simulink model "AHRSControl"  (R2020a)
settings: Solver=FixedStepDiscrete  StartTime=0.0  StopTime=10.0  FixedStep=0.01  RelTol=1e-3  EnableMultiTasking=on
model workspace (MAT data in the model file):
  Ts : Simulink.Parameter (value not decoded)
symbols that are objects in the model workspace (value not decoded): Ts
undefined symbols (not defined in the file or in its folder): DiscIntNeverNeededParam
libraries: simulink x3, HeliLibrary_New x3

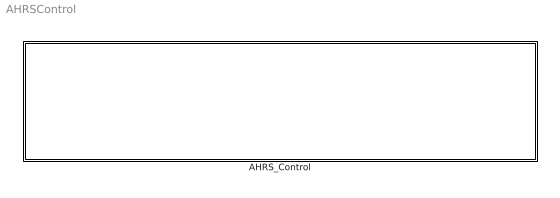
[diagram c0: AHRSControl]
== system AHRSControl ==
  AHRS_Control : Subsystem  TreatAsAtomicUnit=on

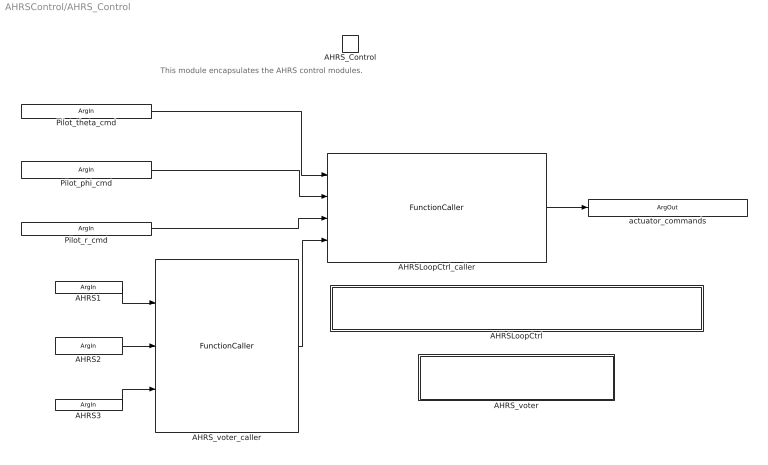
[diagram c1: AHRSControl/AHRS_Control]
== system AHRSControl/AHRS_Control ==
  note: This module encapsulates the AHRS control modules.
  AHRS_Control : TriggerPort  TriggerType=function-call  IsSimulinkFunction=on  FunctionName=AHRS_Control  FunctionVisibility=scoped  VariantControl=Variant  PortDimensions=1
  AHRSLoopCtrl : Subsystem  TreatAsAtomicUnit=on
  AHRSLoopCtrl_caller : FunctionCaller  FunctionPrototype=actuator_commands = AHRSLoopCtrl(Pilot_theta_cmd,Pilot_phi_cmd,Pilot_r_cmd,voted_fb)
  AHRS_voter : Subsystem  TreatAsAtomicUnit=on
  AHRS_voter_caller : FunctionCaller  FunctionPrototype=voted_fb = AHRS_voter(AHRS1,AHRS2,AHRS3)
  Pilot_theta_cmd : ArgIn  OutMin=-32768  OutMax=32767  OutDataTypeStr=int16  ArgumentName=Pilot_theta_cmd
  Pilot_phi_cmd : ArgIn  Port=2  OutMin=-32768  OutMax=32767  OutDataTypeStr=int16  ArgumentName=Pilot_phi_cmd
  Pilot_r_cmd : ArgIn  Port=3  OutMin=-32768  OutMax=32767  OutDataTypeStr=int16  ArgumentName=Pilot_r_cmd
  AHRS1 : ArgIn  Port=4  OutDataTypeStr=Bus: AHRS_Bus  ArgumentName=AHRS1
  AHRS2 : ArgIn  Port=5  OutDataTypeStr=Bus: AHRS_Bus  ArgumentName=AHRS2
  AHRS3 : ArgIn  Port=6  OutDataTypeStr=Bus: AHRS_Bus  ArgumentName=AHRS3
  actuator_commands : ArgOut  PortDimensions=3  ArgumentName=actuator_commands
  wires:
  AHRS3/1 -> AHRS_voter_caller/3
  AHRS1/1 -> AHRS_voter_caller/1
  AHRS2/1 -> AHRS_voter_caller/2
  Pilot_theta_cmd/1 -> AHRSLoopCtrl_caller/1
  Pilot_r_cmd/1 -> AHRSLoopCtrl_caller/3
  AHRS_voter_caller/1 -> AHRSLoopCtrl_caller/4
  AHRSLoopCtrl_caller/1 -> actuator_commands/1
  Pilot_phi_cmd/1 -> AHRSLoopCtrl_caller/2

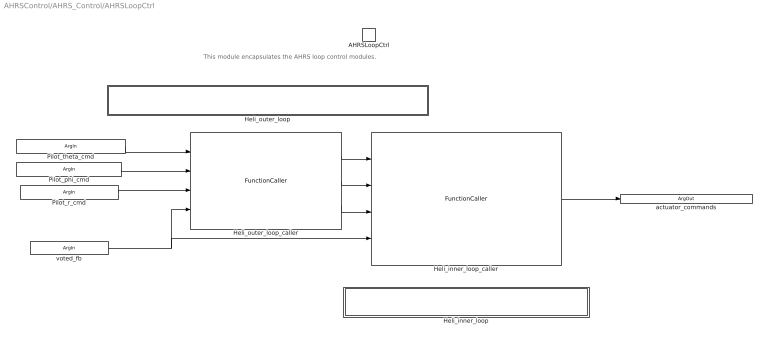
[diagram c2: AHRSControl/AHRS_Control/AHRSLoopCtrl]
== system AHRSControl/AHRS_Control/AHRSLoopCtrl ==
  note: This module encapsulates the AHRS loop control modules.
  AHRSLoopCtrl : TriggerPort  TriggerType=function-call  IsSimulinkFunction=on  FunctionName=AHRSLoopCtrl  FunctionVisibility=scoped  VariantControl=Variant  PortDimensions=1
  Heli_inner_loop : Subsystem  TreatAsAtomicUnit=on
  Heli_inner_loop_caller : FunctionCaller  FunctionPrototype=actuator_commands = Heli_inner_loop(theta_cmd,phi_cmd,r_cmd,voted_fb)
  Heli_outer_loop : Subsystem  TreatAsAtomicUnit=on
  Heli_outer_loop_caller : FunctionCaller  FunctionPrototype=[theta_cmd,phi_cmd,r_cmd] = Heli_outer_loop(Pilot_theta_cmd,Pilot_phi_cmd,Pilot_r_cmd,voted_fb)
  Pilot_theta_cmd : ArgIn  OutMin=-32768  OutMax=32767  OutDataTypeStr=int16  ArgumentName=Pilot_theta_cmd
  Pilot_phi_cmd : ArgIn  Port=2  OutMin=-32768  OutMax=32767  OutDataTypeStr=int16  ArgumentName=Pilot_phi_cmd
  Pilot_r_cmd : ArgIn  Port=3  OutMin=-32768  OutMax=32767  OutDataTypeStr=int16  ArgumentName=Pilot_r_cmd
  voted_fb : ArgIn  Port=4  OutMin=-180  OutMax=180  PortDimensions=5  ArgumentName=voted_fb
  actuator_commands : ArgOut  PortDimensions=3  ArgumentName=actuator_commands
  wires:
  Pilot_phi_cmd/1 -> Heli_outer_loop_caller/2
  Heli_outer_loop_caller/3 -> Heli_inner_loop_caller/3
  Heli_outer_loop_caller/1 -> Heli_inner_loop_caller/1
  Heli_inner_loop_caller/1 -> actuator_commands/1
  Heli_outer_loop_caller/2 -> Heli_inner_loop_caller/2
  voted_fb/1 -> Heli_outer_loop_caller/4, Heli_inner_loop_caller/4
  Pilot_r_cmd/1 -> Heli_outer_loop_caller/3
  Pilot_theta_cmd/1 -> Heli_outer_loop_caller/1

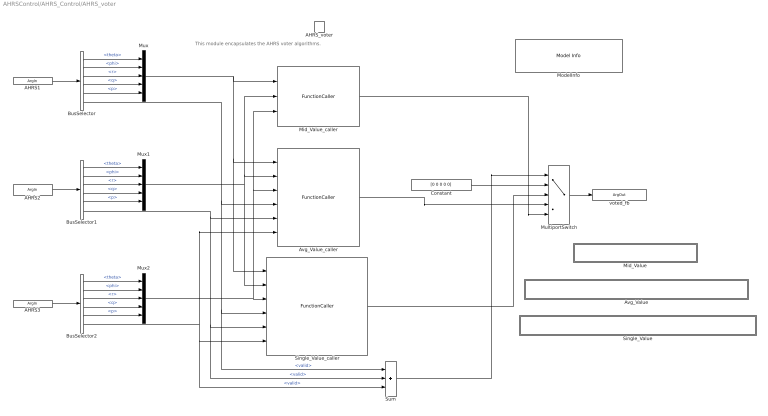
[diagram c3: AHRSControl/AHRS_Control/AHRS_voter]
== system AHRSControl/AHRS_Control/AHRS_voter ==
  note: This module encapsulates the AHRS voter algorithms.
  AHRS_voter : TriggerPort  TriggerType=function-call  IsSimulinkFunction=on  FunctionName=AHRS_voter  FunctionVisibility=scoped  VariantControl=Variant  PortDimensions=1
  Avg_Value : Subsystem  TreatAsAtomicUnit=on  RTWFcnName=Avg_Value
  Avg_Value_caller : FunctionCaller  FunctionPrototype=Avg_Value = Avg_Value(AHRS1,AHRS2,AHRS3,AHRS1_Valid,AHRS2_Valid,AHRS3_Valid)
  BusSelector : BusSelector  OutputSignals=theta,phi,r,q,p,valid
  BusSelector1 : BusSelector  OutputSignals=theta,phi,r,q,p,valid
  BusSelector2 : BusSelector  OutputSignals=theta,phi,r,q,p,valid
  Constant : Constant  Value=[0 0 0 0 0]
  Mid_Value : Subsystem  TreatAsAtomicUnit=on  RTWFcnName=Mid_Value
  Mid_Value_caller : FunctionCaller  FunctionPrototype=Mid_Value = Mid_Value(AHRS1,AHRS2,AHRS3)
  ModelInfo : simulink/Model-Wide Utilities/Model Info  Frame=on  DisplayStringWithTags=|  HorizontalTextAlignment=Center  LeftAlignmentValue=0.5
      | Model Name: %<ModelName>
      | Model Version: %<ModelVersion>
      | Last Modified: %<LastModificationDate>
      | 
      | Copyright 2016 The MathWorks, Inc.
  MultiportSwitch : MultiPortSwitch  DataPortOrder=Zero-based contiguous  Inputs=4  DiagnosticForDefault=None  zeroidx=on
  Mux : Mux  Inputs=5
  Mux1 : Mux  Inputs=5
  Mux2 : Mux  Inputs=5
  Single_Value : Subsystem  TreatAsAtomicUnit=on  RTWFcnName=Single_Value
  Single_Value_caller : FunctionCaller  FunctionPrototype=Single_Value = Single_Value(AHRS1,AHRS2,AHRS3,AHRS1_Valid,AHRS2_Valid,AHRS3_Valid)
  Sum : Sum  Inputs=+++  OutDataTypeStr=uint32
  AHRS1 : ArgIn  OutDataTypeStr=Bus: AHRS_Bus  ArgumentName=AHRS1
  AHRS2 : ArgIn  Port=2  OutDataTypeStr=Bus: AHRS_Bus  ArgumentName=AHRS2
  AHRS3 : ArgIn  Port=3  OutDataTypeStr=Bus: AHRS_Bus  ArgumentName=AHRS3
  voted_fb : ArgOut  OutMin=-180  OutMax=180  PortDimensions=5  ArgumentName=voted_fb
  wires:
  BusSelector2/5 -> Mux2/5  "<p>"
  Mux2/1 -> Avg_Value_caller/3, Mid_Value_caller/3, Single_Value_caller/3
  BusSelector/4 -> Mux/4  "<q>"
  BusSelector2/1 -> Mux2/1  "<theta>"
  AHRS3/1 -> BusSelector2/1
  BusSelector/2 -> Mux/2  "<phi>"
  BusSelector2/2 -> Mux2/2  "<phi>"
  BusSelector2/3 -> Mux2/3  "<r>"
  BusSelector1/2 -> Mux1/2  "<phi>"
  Sum/1 -> MultiportSwitch/1
  BusSelector1/4 -> Mux1/4  "<q>"
  Constant/1 -> MultiportSwitch/2
  BusSelector2/4 -> Mux2/4  "<q>"
  BusSelector2/6 -> Sum/3, Single_Value_caller/6, Avg_Value_caller/6  "<valid>"
  BusSelector/6 -> Sum/1, Single_Value_caller/4, Avg_Value_caller/4  "<valid>"
  BusSelector1/3 -> Mux1/3  "<r>"
  BusSelector/1 -> Mux/1  "<theta>"
  Mux/1 -> Mid_Value_caller/1, Single_Value_caller/1, Avg_Value_caller/1
  AHRS2/1 -> BusSelector1/1
  BusSelector/3 -> Mux/3  "<r>"
  Single_Value_caller/1 -> MultiportSwitch/3
  BusSelector1/1 -> Mux1/1  "<theta>"
  BusSelector1/5 -> Mux1/5  "<p>"
  Mux1/1 -> Single_Value_caller/2, Avg_Value_caller/2, Mid_Value_caller/2
  BusSelector/5 -> Mux/5  "<p>"
  MultiportSwitch/1 -> voted_fb/1
  AHRS1/1 -> BusSelector/1
  Mid_Value_caller/1 -> MultiportSwitch/5
  Avg_Value_caller/1 -> MultiportSwitch/4
  BusSelector1/6 -> Sum/2, Single_Value_caller/5, Avg_Value_caller/5  "<valid>"

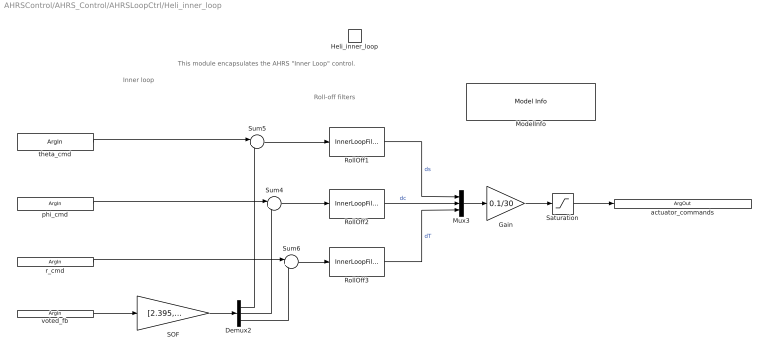
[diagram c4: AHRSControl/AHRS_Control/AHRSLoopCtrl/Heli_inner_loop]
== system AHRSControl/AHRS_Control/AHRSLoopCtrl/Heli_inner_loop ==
  note: This module encapsulates the AHRS "Inner Loop" control.
  note: Roll-off filters
  note: Inner loop
  Heli_inner_loop : TriggerPort  TriggerType=function-call  IsSimulinkFunction=on  FunctionName=Heli_inner_loop  FunctionVisibility=scoped  VariantControl=Variant  PortDimensions=1
  Demux2 : Demux  Outputs=3
  Gain : Gain  Gain=0.1/30
  ModelInfo : simulink/Model-Wide Utilities/Model Info  Frame=on  DisplayStringWithTags=|  HorizontalTextAlignment=Center  LeftAlignmentValue=0.5
      | Model Name: %<ModelName>
      | Model Version: %<ModelVersion>
      | Last Modified: %<LastModificationDate>
      | 
      | Copyright 2016 The MathWorks, Inc.
  Mux3 : Mux  Inputs=3
  RollOff1 : HeliLibrary_New/InnerLoopFilter  Tag=FilterWizardSubSystem  RequirementInfo={} %GIDa_ac7f675d_0c04_474f_b6aa_16ea1999b46b  SystemSampleTime=-1  Latency=0  AutoFrameSizeCalculation=off
  RollOff2 : HeliLibrary_New/InnerLoopFilter  Tag=FilterWizardSubSystem  SystemSampleTime=-1  Latency=0  AutoFrameSizeCalculation=off
  RollOff3 : HeliLibrary_New/InnerLoopFilter  Tag=FilterWizardSubSystem  SystemSampleTime=-1  Latency=0  AutoFrameSizeCalculation=off
  SOF : Gain  Gain=[2.395, -0.3609, -0.002145, 0.8087, -0.0205; -0.1427, -1.115, 0.04573, -0.04318, -0.1007; -0.02792, -0.02229, -2.025, -0.06152, 0.03151;]  Multiplication=Matrix(K*u) (u vector)
  Saturation : Saturate  UpperLimit=0.1  LowerLimit=-0.1
  Sum4 : Sum  Inputs=|+-
  Sum5 : Sum  Inputs=|+-
  Sum6 : Sum  Inputs=|+-
  theta_cmd : ArgIn  OutMin=-30  OutMax=30  ArgumentName=theta_cmd
  phi_cmd : ArgIn  Port=2  OutMin=-30  OutMax=30  ArgumentName=phi_cmd
  r_cmd : ArgIn  Port=3  OutMin=-30  OutMax=30  ArgumentName=r_cmd
  voted_fb : ArgIn  Port=4  OutMin=-180  OutMax=180  PortDimensions=5  ArgumentName=voted_fb
  actuator_commands : ArgOut  PortDimensions=3  ArgumentName=actuator_commands
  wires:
  Demux2/3 -> Sum6/2
  voted_fb/1 -> SOF/1
  Saturation/1 -> actuator_commands/1
  r_cmd/1 -> Sum6/1
  Demux2/1 -> Sum5/2
  Demux2/2 -> Sum4/2
  RollOff1/1 -> Mux3/1  "ds"
  RollOff3/1 -> Mux3/3  "dT"
  theta_cmd/1 -> Sum5/1
  Gain/1 -> Saturation/1
  Sum5/1 -> RollOff1/1
  RollOff2/1 -> Mux3/2  "dc"
  SOF/1 -> Demux2/1
  Mux3/1 -> Gain/1
  Sum6/1 -> RollOff3/1
  Sum4/1 -> RollOff2/1
  phi_cmd/1 -> Sum4/1

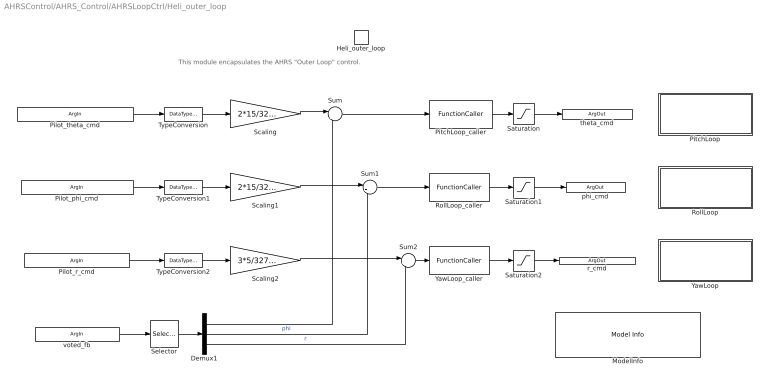
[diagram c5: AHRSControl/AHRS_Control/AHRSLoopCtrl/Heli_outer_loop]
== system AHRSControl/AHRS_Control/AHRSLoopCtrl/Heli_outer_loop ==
  note: This module encapsulates the AHRS "Outer Loop" control.
  Heli_outer_loop : TriggerPort  TriggerType=function-call  IsSimulinkFunction=on  FunctionName=Heli_outer_loop  FunctionVisibility=scoped  VariantControl=Variant  PortDimensions=1
  Demux1 : Demux  Outputs=3
  ModelInfo : simulink/Model-Wide Utilities/Model Info  Frame=on  DisplayStringWithTags=|  HorizontalTextAlignment=Center  LeftAlignmentValue=0.5
      | Model Name: %<ModelName>
      | Model Version: %<ModelVersion>
      | Last Modified: %<LastModificationDate>
      | 
      | Copyright 2016 The MathWorks, Inc.
  PitchLoop : Subsystem  TreatAsAtomicUnit=on
  PitchLoop_caller : FunctionCaller  FunctionPrototype=Y = PitchLoop(U)  InputArgumentSpecifications=double(1)  OutputArgumentSpecifications=double(1)
  RollLoop : Subsystem  TreatAsAtomicUnit=on
  RollLoop_caller : FunctionCaller  FunctionPrototype=Y = RollLoop(U)  InputArgumentSpecifications=double(1)  OutputArgumentSpecifications=double(1)
  Saturation : Saturate  UpperLimit=30  LowerLimit=-30
  Saturation1 : Saturate  UpperLimit=30  LowerLimit=-30
  Saturation2 : Saturate  UpperLimit=30  LowerLimit=-30
  Scaling : Gain  Gain=2*15/32767
  Scaling1 : Gain  Gain=2*15/32767
  Scaling2 : Gain  Gain=3*5/32767
  Selector : Selector  InputPortWidth=5  IndexOptions=Index vector (dialog)  Indices=[1 2 3]  OutputSizes=1
  Sum : Sum  Inputs=|+-  InputSameDT=on
  Sum1 : Sum  Inputs=|+-  InputSameDT=on
  Sum2 : Sum  Inputs=|+-  InputSameDT=on
  TypeConversion : DataTypeConversion  OutDataTypeStr=double
  TypeConversion1 : DataTypeConversion  OutDataTypeStr=double
  TypeConversion2 : DataTypeConversion  OutDataTypeStr=double
  YawLoop : Subsystem  TreatAsAtomicUnit=on
  YawLoop_caller : FunctionCaller  FunctionPrototype=Y = YawLoop(U)  InputArgumentSpecifications=double(1)  OutputArgumentSpecifications=double(1)
  Pilot_theta_cmd : ArgIn  OutMin=-32768  OutMax=32767  OutDataTypeStr=int16  ArgumentName=Pilot_theta_cmd
  Pilot_phi_cmd : ArgIn  Port=2  OutMin=-32768  OutMax=32767  OutDataTypeStr=int16  ArgumentName=Pilot_phi_cmd
  Pilot_r_cmd : ArgIn  Port=3  OutMin=-32768  OutMax=32767  OutDataTypeStr=int16  ArgumentName=Pilot_r_cmd
  voted_fb : ArgIn  Port=4  OutMin=-180  OutMax=180  PortDimensions=5  ArgumentName=voted_fb
  theta_cmd : ArgOut  OutMin=-30  OutMax=30  ArgumentName=theta_cmd
  phi_cmd : ArgOut  Port=2  OutMin=-30  OutMax=30  ArgumentName=phi_cmd
  r_cmd : ArgOut  Port=3  OutMin=-30  OutMax=30  ArgumentName=r_cmd
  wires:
  Selector/1 -> Demux1/1
  Scaling2/1 -> Sum2/1
  Scaling1/1 -> Sum1/1
  TypeConversion2/1 -> Scaling2/1
  Pilot_r_cmd/1 -> TypeConversion2/1
  Demux1/3 -> Sum2/2  "r"
  Pilot_phi_cmd/1 -> TypeConversion1/1
  Demux1/2 -> Sum1/2  "phi"
  Saturation1/1 -> phi_cmd/1
  TypeConversion1/1 -> Scaling1/1
  Saturation2/1 -> r_cmd/1
  voted_fb/1 -> Selector/1
  Sum1/1 -> RollLoop_caller/1
  RollLoop_caller/1 -> Saturation1/1
  Sum2/1 -> YawLoop_caller/1
  YawLoop_caller/1 -> Saturation2/1
  TypeConversion/1 -> Scaling/1
  PitchLoop_caller/1 -> Saturation/1
  Saturation/1 -> theta_cmd/1
  Sum/1 -> PitchLoop_caller/1
  Demux1/1 -> Sum/2
  Pilot_theta_cmd/1 -> TypeConversion/1
  Scaling/1 -> Sum/1

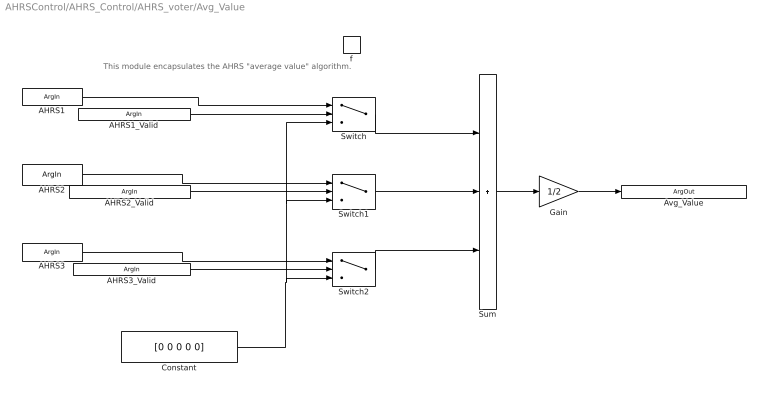
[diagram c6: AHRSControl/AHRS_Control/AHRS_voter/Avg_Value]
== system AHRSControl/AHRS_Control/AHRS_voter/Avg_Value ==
  note: This module encapsulates the AHRS "average value" algorithm.
  f : TriggerPort  TriggerType=function-call  IsSimulinkFunction=on  FunctionName=Avg_Value  FunctionVisibility=scoped  VariantControl=Variant  PortDimensions=1
  Constant : Constant  Value=[0 0 0 0 0]
  Gain : Gain  Gain=1/2
  Sum : Sum  Inputs=+++
  Switch : Switch  Criteria=u2 ~= 0
  Switch1 : Switch  Criteria=u2 ~= 0
  Switch2 : Switch  Criteria=u2 ~= 0
  AHRS1 : ArgIn  PortDimensions=5  ArgumentName=AHRS1
  AHRS2 : ArgIn  Port=2  PortDimensions=5  ArgumentName=AHRS2
  AHRS3 : ArgIn  Port=3  PortDimensions=5  ArgumentName=AHRS3
  AHRS1_Valid : ArgIn  Port=4  OutDataTypeStr=boolean  ArgumentName=AHRS1_Valid
  AHRS2_Valid : ArgIn  Port=5  OutDataTypeStr=boolean  ArgumentName=AHRS2_Valid
  AHRS3_Valid : ArgIn  Port=6  OutDataTypeStr=boolean  ArgumentName=AHRS3_Valid
  Avg_Value : ArgOut  PortDimensions=5  ArgumentName=Avg_Value
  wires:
  Gain/1 -> Avg_Value/1
  Sum/1 -> Gain/1
  AHRS1_Valid/1 -> Switch/2
  AHRS1/1 -> Switch/1
  Switch/1 -> Sum/1
  Switch1/1 -> Sum/2
  Switch2/1 -> Sum/3
  AHRS2_Valid/1 -> Switch1/2
  AHRS3_Valid/1 -> Switch2/2
  AHRS2/1 -> Switch1/1
  AHRS3/1 -> Switch2/1
  Constant/1 -> Switch/3, Switch1/3, Switch2/3

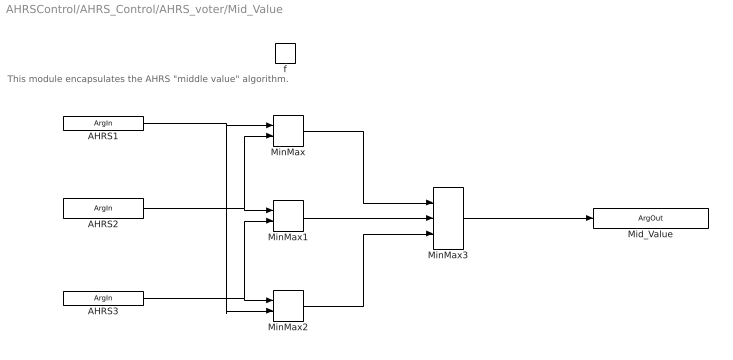
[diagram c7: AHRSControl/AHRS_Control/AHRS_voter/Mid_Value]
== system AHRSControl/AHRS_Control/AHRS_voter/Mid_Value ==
  note: This module encapsulates the AHRS "middle value" algorithm.
  f : TriggerPort  TriggerType=function-call  IsSimulinkFunction=on  FunctionName=Mid_Value  FunctionVisibility=scoped  VariantControl=Variant  PortDimensions=1
  MinMax : MinMax  Inputs=2
  MinMax1 : MinMax  Inputs=2
  MinMax2 : MinMax  Inputs=2
  MinMax3 : MinMax  Function=max  Inputs=3
  AHRS1 : ArgIn  PortDimensions=5  ArgumentName=AHRS1
  AHRS2 : ArgIn  Port=2  PortDimensions=5  ArgumentName=AHRS2
  AHRS3 : ArgIn  Port=3  PortDimensions=5  ArgumentName=AHRS3
  Mid_Value : ArgOut  PortDimensions=5  ArgumentName=Mid_Value
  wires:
  AHRS1/1 -> MinMax2/2, MinMax/1
  AHRS3/1 -> MinMax1/2, MinMax2/1
  AHRS2/1 -> MinMax/2, MinMax1/1
  MinMax1/1 -> MinMax3/2
  MinMax/1 -> MinMax3/1
  MinMax2/1 -> MinMax3/3
  MinMax3/1 -> Mid_Value/1

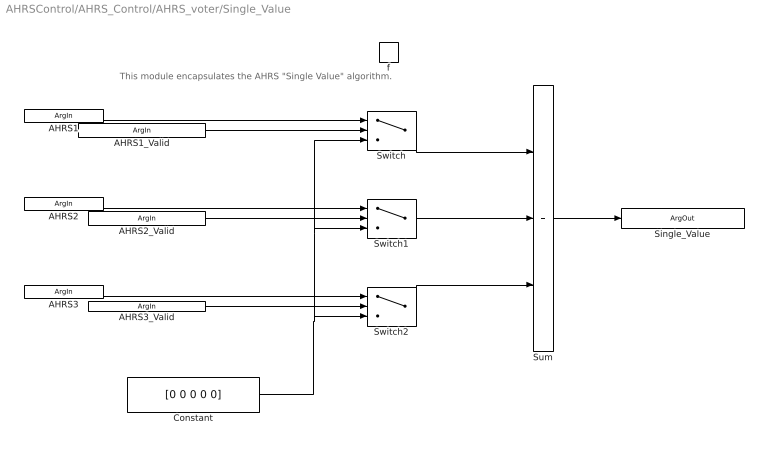
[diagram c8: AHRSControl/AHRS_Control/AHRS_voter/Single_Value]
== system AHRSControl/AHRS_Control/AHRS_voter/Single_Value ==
  note: This module encapsulates the AHRS "Single Value" algorithm.
  f : TriggerPort  TriggerType=function-call  IsSimulinkFunction=on  FunctionName=Single_Value  FunctionVisibility=scoped  VariantControl=Variant  PortDimensions=1
  Constant : Constant  Value=[0 0 0 0 0]
  Sum : Sum  Inputs=+++
  Switch : Switch  Criteria=u2 ~= 0
  Switch1 : Switch  Criteria=u2 ~= 0
  Switch2 : Switch  Criteria=u2 ~= 0
  AHRS1 : ArgIn  PortDimensions=5  ArgumentName=AHRS1
  AHRS2 : ArgIn  Port=2  PortDimensions=5  ArgumentName=AHRS2
  AHRS3 : ArgIn  Port=3  PortDimensions=5  ArgumentName=AHRS3
  AHRS1_Valid : ArgIn  Port=4  OutDataTypeStr=boolean  ArgumentName=AHRS1_Valid
  AHRS2_Valid : ArgIn  Port=5  OutDataTypeStr=boolean  ArgumentName=AHRS2_Valid
  AHRS3_Valid : ArgIn  Port=6  OutDataTypeStr=boolean  ArgumentName=AHRS3_Valid
  Single_Value : ArgOut  PortDimensions=5  ArgumentName=Single_Value
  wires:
  Constant/1 -> Switch2/3, Switch1/3, Switch/3
  AHRS3/1 -> Switch2/1
  AHRS2/1 -> Switch1/1
  AHRS3_Valid/1 -> Switch2/2
  AHRS2_Valid/1 -> Switch1/2
  Switch2/1 -> Sum/3
  Switch1/1 -> Sum/2
  Switch/1 -> Sum/1
  AHRS1/1 -> Switch/1
  AHRS1_Valid/1 -> Switch/2
  Sum/1 -> Single_Value/1

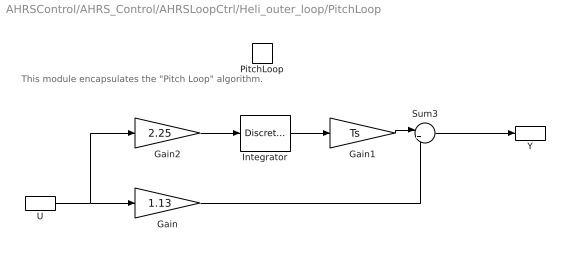
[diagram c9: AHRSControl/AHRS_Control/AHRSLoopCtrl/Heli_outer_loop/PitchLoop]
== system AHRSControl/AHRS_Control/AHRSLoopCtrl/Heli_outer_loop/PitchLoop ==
  note: This module encapsulates the "Pitch Loop" algorithm.
  PitchLoop : TriggerPort  TriggerType=function-call  IsSimulinkFunction=on  FunctionName=PitchLoop  FunctionVisibility=scoped  VariantControl=Variant  PortDimensions=1
  Gain : Gain  Gain=1.13
  Gain1 : Gain  Gain=Ts
  Gain2 : Gain  Gain=2.25
  Integrator : DiscreteIntegrator  IntegratorMethod=Accumulation: Forward Euler  SampleTime=-1  LimitOutput=on  UpperSaturationLimit=10  LowerSaturationLimit=-10  ICPrevOutput=DiscIntNeverNeededParam  ICPrevScaledInput=DiscIntNeverNeededParam
  Sum3 : Sum  Inputs=|++
  U : ArgIn  ArgumentName=U
  Y : ArgOut  ArgumentName=Y
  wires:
  Gain2/1 -> Integrator/1
  Sum3/1 -> Y/1
  Integrator/1 -> Gain1/1
  U/1 -> Gain/1, Gain2/1
  Gain/1 -> Sum3/2
  Gain1/1 -> Sum3/1

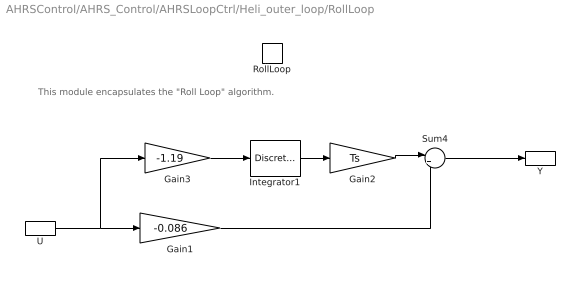
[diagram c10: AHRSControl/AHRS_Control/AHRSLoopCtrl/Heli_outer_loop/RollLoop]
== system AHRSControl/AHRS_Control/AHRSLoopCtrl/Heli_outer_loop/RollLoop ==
  note: This module encapsulates the "Roll Loop" algorithm.
  RollLoop : TriggerPort  TriggerType=function-call  IsSimulinkFunction=on  FunctionName=RollLoop  FunctionVisibility=scoped  VariantControl=Variant  PortDimensions=1
  Gain1 : Gain  Gain=-0.086
  Gain2 : Gain  Gain=Ts
  Gain3 : Gain  Gain=-1.19
  Integrator1 : DiscreteIntegrator  IntegratorMethod=Accumulation: Forward Euler  SampleTime=-1  LimitOutput=on  UpperSaturationLimit=10  LowerSaturationLimit=-10  ICPrevOutput=DiscIntNeverNeededParam  ICPrevScaledInput=DiscIntNeverNeededParam
  Sum4 : Sum  Inputs=|++
  U : ArgIn  ArgumentName=U
  Y : ArgOut  ArgumentName=Y
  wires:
  Sum4/1 -> Y/1
  Gain3/1 -> Integrator1/1
  Gain1/1 -> Sum4/2
  Integrator1/1 -> Gain2/1
  U/1 -> Gain3/1, Gain1/1
  Gain2/1 -> Sum4/1

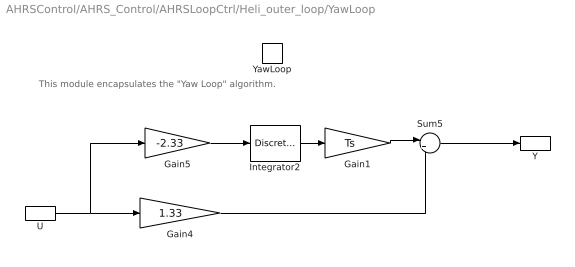
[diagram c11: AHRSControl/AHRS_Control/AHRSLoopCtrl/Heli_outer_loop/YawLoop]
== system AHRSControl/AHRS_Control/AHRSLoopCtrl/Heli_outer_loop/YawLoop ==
  note: This module encapsulates the "Yaw Loop" algorithm.
  YawLoop : TriggerPort  TriggerType=function-call  IsSimulinkFunction=on  FunctionName=YawLoop  FunctionVisibility=scoped  VariantControl=Variant  PortDimensions=1
  Gain1 : Gain  Gain=Ts
  Gain4 : Gain  Gain=1.33
  Gain5 : Gain  Gain=-2.33
  Integrator2 : DiscreteIntegrator  IntegratorMethod=Accumulation: Forward Euler  SampleTime=-1  LimitOutput=on  UpperSaturationLimit=10  LowerSaturationLimit=-10  ICPrevOutput=DiscIntNeverNeededParam  ICPrevScaledInput=DiscIntNeverNeededParam
  Sum5 : Sum  Inputs=|++
  U : ArgIn  ArgumentName=U
  Y : ArgOut  ArgumentName=Y
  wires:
  Integrator2/1 -> Gain1/1
  U/1 -> Gain5/1, Gain4/1
  Gain4/1 -> Sum5/2
  Gain5/1 -> Integrator2/1
  Sum5/1 -> Y/1
  Gain1/1 -> Sum5/1
